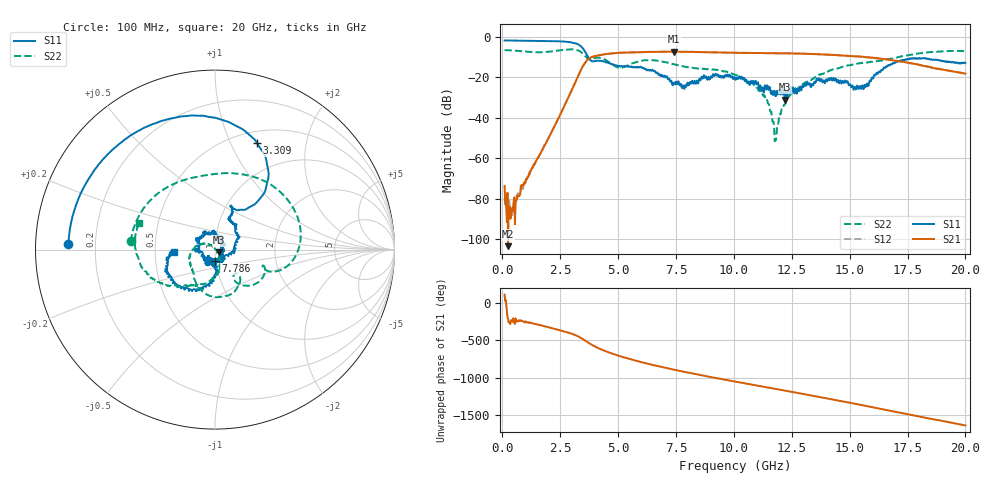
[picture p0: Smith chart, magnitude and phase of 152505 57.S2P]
!  2-Port S-parameters saved by WinCal
! VAR MeasName=S-Parameters (CALIBRATED_DATA) read from VNA (N5230C)
! VAR MeasDate=4/10/2015 9:34:31 AM
! VAR NAME=152505 57
! VAR FILENAME=152505 57.S2P
! VAR DATE=4/10/2015 9:34:31 AM
! VAR PHYS_PORTS=1,2
# Hz S DB R 50
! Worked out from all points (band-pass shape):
!   801 points, 100 MHz to 20 GHz, reference 50 ohm
!   highest |S21| = -7.29 dB at 7.413 GHz (marker M1); lowest = -103.3 dB at 249.2 MHz (marker M2)
!   |S21| within 3 dB of the highest: 3.806 GHz to 16.01 GHz (12.2 GHz wide, 123 % of centre)
!   lowest |S11| = -31.0 dB at 12.21 GHz (marker M3), VSWR 1.06, Z = 52.4 - j1.52 ohm
!   |S11| at or under -10 dB: 3.712 GHz to end of sweep
!   |S22| runs from -51.5 to -6.1 dB; largest |S21 - S12| = 0.0059
!   S11 on the Smith chart (normalised r, x): 100 MHz: 0.10, +0.02; 3.309 GHz: 0.63, +1.26; 7.786 GHz: 1.00, -0.13; 20 GHz: 0.63, -0.02
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1e8  -1.75 177.6  -73.59 113.6  -79.56 -11.9  -6.54 174.4
2.4925e8  -1.75 174.1  -103.33 152.9  -84.54 149.8  -6.57 165.9
6.72125e8  -1.79 164.0  -78.73 113.5  -77.15 125.0  -6.87 142.7
2.164625e9  -2.06 123.9  -46.17 22.7  -46.22 21.7  -7.11 73.9
3.308875e9  -3.88 68.6  -18.37 -92.0  -18.43 -92.1  -6.83 -3.3
3.43325e9  -5.07 58.8  -15.46 -113.7  -15.50 -113.6  -7.78 -13.7
3.856125e9  -11.95 60.1  -10.00 162.3  -10.05 162.3  -10.93 -18.4
4.353625e9  -12.06 68.2  -8.70 88.8  -8.74 88.5  -10.75 -42.4
5.22425e9  -14.59 64.4  -7.76 -5.2  -7.79 -5.1  -14.98 -48.2
6.741625e9  -18.61 17.7  -7.35 -125.9  -7.37 -126.1  -11.84 -99.0
7.41325e9  -22.57 -41.4  -7.29 -171.9  -7.30 -171.8  -13.52 -120.4
7.786375e9  -24.05 -88.0  -7.34 163.5  -7.35 163.8  -14.44 -129.2
8.880875e9  -20.61 166.8  -7.55 95.8  -7.56 96.1  -15.94 -149.7
1.005e10  -20.36 111.4  -7.81 28.5  -7.85 28.5  -18.74 176.3
1.13435e10  -23.87 29.7  -7.99 -44.0  -8.01 -43.7  -29.55 131.0
1.179125e10  -29.23 14.4  -8.03 -68.7  -8.03 -68.9  -51.26 31.2
1.221412e10  -31.02 -31.1  -8.12 -92.8  -8.09 -93.2  -33.26 -59.7
1.338325e10  -23.22 -82.4  -8.44 -159.8  -8.40 -159.6  -20.74 -73.7
1.5025e10  -23.46 -129.4  -9.44 104.0  -9.47 104.0  -13.86 -108.3
1.669162e10  -13.75 -98.8  -11.27 2.4  -11.22 2.1  -10.88 -133.4
1.796025e10  -10.86 -148.2  -13.64 -76.6  -13.73 -76.0  -8.13 -156.3
2e10  -12.84 -177.1  -18.12 161.3  -18.07 161.5  -6.98 160.6
